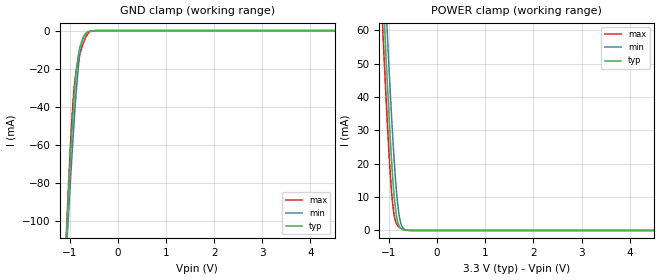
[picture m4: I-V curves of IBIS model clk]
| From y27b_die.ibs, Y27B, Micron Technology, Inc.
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|   clk MODEL
[Model]   clk
Model_type   Input
Vinl = 800.000mV
Vinh = 2.000V
|   typ   min   max
C_comp   2.100pF   1.850pF   2.350pF
[Voltage Range]   3.300V   3.000V   3.600V
| Junction Temperature (Ambient temp is 25C typ, 70C min, 0C max)
[Temperature Range]   40.0   85.0   0.0
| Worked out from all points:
|   GND clamp passes 1 mA (typ) near -0.64 V on its own axis
|   POWER clamp passes 1 mA (typ) near -0.77 V on its own axis
[GND Clamp]
|   Voltage   I(typ)   I(min)   I(max)
-3.3V     -1.431A    -1.275A    -1.646A
-1.07V    -109mA     -116.8mA   -106mA
-1.05V    -98.79mA   -107.6mA   -94.47mA
-990mV    -69.48mA   -80.79mA   -62.28mA
-950mV    -51.55mA   -63.83mA   -44.07mA
-910mV    -35.7mA    -47.9mA    -30.18mA
-850mV    -18.03mA   -27.05mA   -18.55mA
-790mV    -8.784mA   -12.06mA   -12.42mA
-750mV    -5.487mA   -6.201mA   -9.085mA
-690mV    -2.425mA   -2.143mA   -4.761mA
-610mV    -575.3uA   -540.4uA   -1.197mA
6.6V      0A         0A         0A
[POWER Clamp]
|   Voltage   I(typ)   I(min)   I(max)
-3.3V     840.5mA    849.5mA    834.5mA
-1.13V    73.22mA    88.26mA    60.66mA
-1.09V    60.82mA    75.77mA    48.38mA
-1.05V    48.83mA    63.59mA    36.68mA
-1.03V    43.05mA    57.65mA    31.13mA
-950mV    21.99mA    35.23mA    12.36mA
-910mV    13.47mA    25.22mA    6.325mA
-870mV    7.092mA    16.47mA    3.065mA
-830mV    3.228mA    9.474mA    1.654mA
-790mV    1.387mA    4.671mA    1.002mA
-710mV    274.6uA    773.7uA    NA
6.6V      0A         0A         0A
